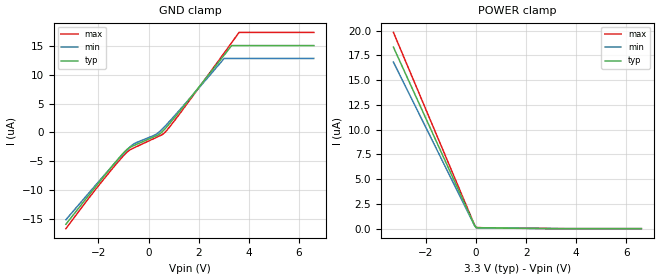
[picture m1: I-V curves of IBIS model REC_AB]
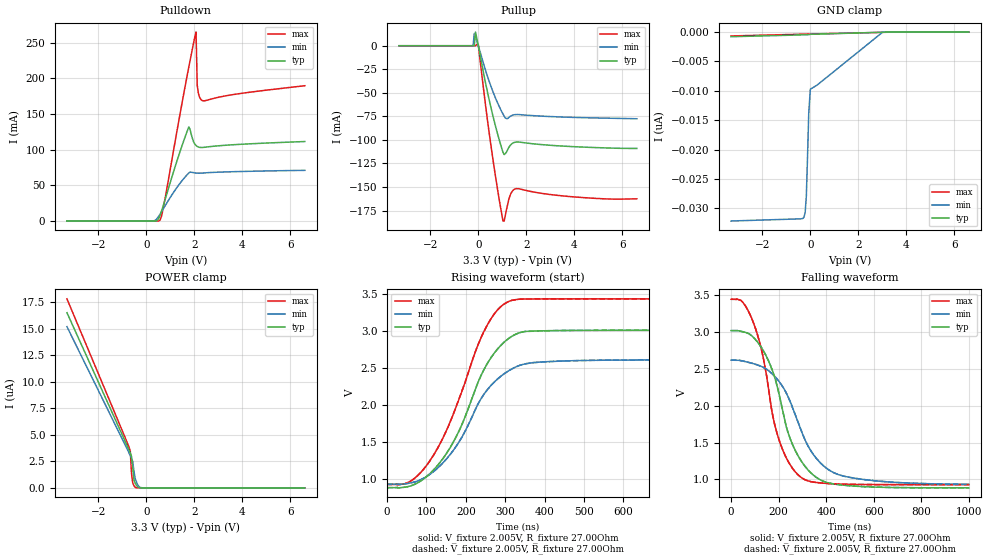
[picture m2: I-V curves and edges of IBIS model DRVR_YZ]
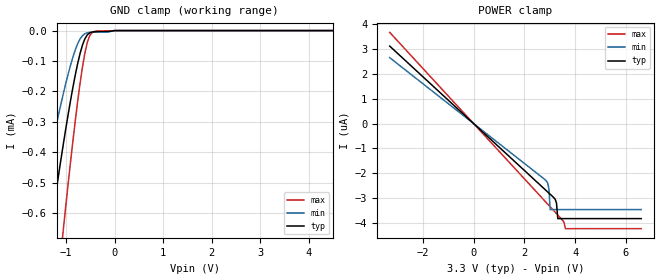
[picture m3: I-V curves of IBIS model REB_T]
| Texas Instruments Incorporated
| ISO35T ISOLATED 3.3V RS-485 TRANSCEIVER with Integrated Transformer Driver
| Marketing part#   Voltage Range   Package-type   #pins/pkg drawing
| ISO35TDW   3.0V - 3.6V   DW   16-pin
| ISO35TDWR   3.0V - 3.6V   DW   16-pin
[IBIS Ver]   4.0
[File name]   iso35t.ibs
[File Rev]   1.2
[Date]   02/28/2011
[Source]   TISPICE Simulations
   Texas Instruments Incorporated.
   Analog-eLab, HPA
   12500 TI Blvd
   Dallas, TX -75243
   For Support e-mail: elab_ibis@list.ti.com
[Notes]   Revision History
   Rev 1.0: 07/08/2008
   - Original model from Data Transmission Products Group
   Rev 1.1: 02/08/2011
   - file name changed from iso35.ibs to iso35_t.ibs
   - Updated header information
   - Updated all models with latest IBIS models generated from TISPICED
   - Pulldown/up non-monotonic warnings reflect true buffer behavior
   in TISPICED
   - Updated ccomp for all models as well
   - D1 and D2 are analog transformer driver pins that are outside
   the scope of IBIS 4.0 and hence are left as NCs
   - All the digtial buffer models are shared between ISO35 and ISO35T
   Rev 1.2: 02/28/2011
   - Removed ISO35 model from the file and renamed the file as ISO35T only
   - DRVR_YZ non-monotonicity is based on original
   simulations in TISPICED
[Disclaimer] This model is designed as an aid for customers of
 Texas Instruments. TI and its licensors and suppliers make no warranties,
 either expressed or implied, with respect to this  model, including the
 warranties of merchantability or fitness for a particular purpose.
 The model is provided solely on an "as is" basis. The entire risk as to
 its quality and performance is with the customer.
[Copyright] (C)Copyright 2011 Texas Instruments Incorporated.
   All rights reserved.
|   ISO35TDW  & ISO35TDWR
[Component]   ISO35TDW
[Manufacturer]  Texas Instruments Incorporated
[Package]   |16-pin DW package
|   typ   min   max
R_pkg   0.04229   0.019   0.0747
L_pkg   1.96583nH   1.3071nH   2.78nH
C_pkg   0.55243pF   0.366pF   0.8774pF
[Pin]   signal_name   model_name   R_pin   L_pin   C_pin
   1   D1   NC   0.01988  2.47032nH   0.87737pF
   2   D2   NC   0.01896  1.75378nH   0.75515pF
   3   GND1   GND   0.01119  1.36813nH   0.62214pF
   4   VCC1   POWER   0.01441  1.13364nH   0.53256pF
   5   R   OUT_R_T 0.02905  1.67358nH   0.55809pF
   6   REN   REB_T   0.03208  1.30711nH   0.39487pF
   7   DE   D_DE_T  0.03561  1.87226nH   0.60690pF
   8   D   D_DE_T  0.03804  2.78001nH   0.80551pF
   9   VCC2   POWER   0.02887  3.18832nH   2.5960pF
   10   GND2   GND   0.06791  2.86161nH   0.65609pF
   11   A   REC_AB  0.07468  2.23033nH   0.39167pF
   12   B   REC_AB  0.06522  2.01365nH   0.38729pF
   13   Z   DRVR_YZ 0.05893  1.87256nH   0.38126pF
   14   Y   DRVR_YZ 0.05043  1.68460nH   0.36601pF
   15   GND2   GND   0.03460  0.66170nH   3.0671pF
   16   GND2   GND   0.02304  3.19116nH   0.88927pF
[Diff_pin]   inv_pin   vdiff   tdelay_typ   tdelay_min   tdelay_max
| The 'A' pin is Diff_pin and the 'B' pin is the inv_pin
11   12   NA   0 0 0
14   13   0.200   0 0 0
[Pin Mapping] pulldown_ref pullup_ref gnd_clamp_ref power_clamp_ref |ext_ref
1   NC   NC
2   NC   NC
3   GND1BUS  NC
4   NC   VCC1BUS
5   GND1BUS  VCC1BUS  GND1BUS  VCC1BUS
6   NC   NC   GND1BUS  VCC1BUS
7   NC   NC   GND1BUS  VCC1BUS
8   NC   NC   GND1BUS  VCC1BUS
9   NC   VCC2BUS
10   GND2BUS  NC
11   NC   NC   GND2BUS  VCC2BUS
12   NC   NC   GND2BUS  VCC2BUS
13   GND2BUS  VCC2BUS  GND2BUS  VCC2BUS
14   GND2BUS  VCC2BUS  GND2BUS  VCC2BUS
15   GND2BUS  NC
16   GND2BUS  NC
| Models and submodels in the file (5): REC_AB (Input), DRVR_YZ (I/O), REB_T (Input), D_DE_T (Input), OUT_R_T (Output)
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|   Receiver Input / Model
[Model]   REC_AB
Model_type   Input
|Signals   A,B
Vinl   = 0.99V
Vinh   = 2.31V
|Rref_diff = 96k  |Input Diff resistance
|Cref_diff = 16pF |Input Diff capacitance
|Vdiff can be +/- 200mV and Common mode can be betweem -7V to 12V
|   typ   min   max
|   (typ PVT)   (Fast PVT)   (Slow PVT)
C_comp   0.2533pF   0.2533pF   0.2533pF
[Model Spec]
Vinl   0.99V   0.9V   1.08V
Vinh   2.31V   2.1V   2.52V
|   typ   min   max
[Temperature Range]   27.0   85   -40
[Voltage range]   3.3V   3.0V   3.6V
[GND Clamp]
|   Voltage   I(typ)   I(min)   I(max)
-3.3V     -15.94uA   -15.15uA   -16.71uA
-2.007V   -8.832uA   -8.611uA   -9.299uA
-912.1mV  -3.159uA   -3.267uA   -3.635uA
-563.8mV  -2.228uA   -1.938uA   -2.639uA
331.7mV   -534.5nA   -236.4nA   -822.3nA
480.9mV   -132.9nA   303.7nA    -516.7nA
679.9mV   743.7nA    1.182uA    128nA
1.327V    4.137uA    4.315uA    3.74uA
3.018V    13.42uA    12.84uA    13.79uA
3.317V    15.08uA    12.84uA    15.58uA
3.615V    15.08uA    12.84uA    17.37uA
6.6V      15.08uA    12.84uA    17.37uA
[POWER Clamp]
|  Voltage   I(typ)   I(min)   I(max)
-3.3V     18.32uA    16.82uA    19.81uA
-66.33mV  368.3nA    338nA      398.3nA
0V        101.5nA    93.2nA     NA
3.615V    0A         0A         0A
6.6V      0A         0A         0A
|   Driver YZ model
[Model]   DRVR_YZ
Model_type   I/O
| Signals   Y,Z
Vinl   = 0.99V
Vinh   = 2.31V
Vmeas   = 2.6V   |Reference voltage for timing measurements
Rref   = 27   |Note: 54 Ohm load; single-ended configuration
Vref   = 2.005V
|   Timing specification test load voltage
|Cref_diff = 50pF
|Rref_diff = 54Ohms
| variable   typ   min   max
| Y/Z  3-state   (typ PVT)   (Slow PVT)   (Fast PVT)
C_comp   30.536pF   30.533pF   31.925pF
| Y/Z high state   (typ PVT)   (Slow PVT)   (Fast PVT)
|C_comp   42.644pF   41.559pF   50.167pF
| Y/Z low state   (typ PVT)   (Fast PVT)   (Slow PVT)
|C_comp   48.779pF   38.475pF   54.688pF
[Model Spec]
Vref   2.005V   1.73V   2.528V
Vmeas   2.6V   2.2V   3.0V
Vinl   0.99V   0.9V   1.08V
Vinh   2.31V   2.1V   2.52V
|   typ   min   max
[Temperature Range]   27.0   85   -40
[Voltage range]   3.3V   3.0V   3.6V
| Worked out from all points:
|   slope of the pulldown table from 0 to 0.495 V, typ, clamps not added: 206 ohm
|   slope of the pullup table from 0 to 0.495 V, typ, clamps not added: 7.93 ohm
|   falling waveform, V_fixture 2.005V, R_fixture 27.00Ohm: 20-80 % time 124ns typ, 150ns min, 100ns max; typ from 3.01 V to 0.886 V
|   rising waveform, V_fixture 2.005V, R_fixture 27.00Ohm: 20-80 % time 111ns typ, 116ns min, 111ns max; typ from 0.886 V to 3.01 V
|   rising waveform, V_fixture 2.005V, R_fixture 27.00Ohm: 20-80 % time 111ns typ, 116ns min, 111ns max; typ from 0.886 V to 3.01 V
|   falling waveform, V_fixture 2.005V, R_fixture 27.00Ohm: 20-80 % time 124ns typ, 150ns min, 100ns max; typ from 3.01 V to 0.886 V
[Pulldown]
|   Voltage   I(typ)   I(min)   I(max)
-3.3V     -1.766pA   -150.1pA   -1.411pA
281.9mV   2.075uA    96.37uA    2.704nA
480.9mV   1.606mA    4.79mA     24.87uA
580.4mV   8.506mA    9.847mA    1.675mA
729.6mV   23.91mA    18.15mA    21.69mA
1.774V    132.1mA    67.49mA    216.4mA
1.973V    110.9mA    67.81mA    250.3mA
2.073V    105.9mA    67.31mA    265.2mA
2.123V    104.6mA    67.17mA    190.6mA
2.222V    103.4mA    67.09mA    173.5mA
2.322V    103.2mA    67.23mA    169.2mA
6.6V      111.5mA    71.11mA    189.8mA
[GND Clamp]
|   Voltage   I(typ)   I(min)   I(max)
-3.3V     -793.9pA   -32.13nA   -666.8pA
-414.6mV  -496.1pA   -31.76nA   -373.8pA
-315.1mV  -485.9pA   -31.7nA    -363.7pA
-265.3mV  -480.7pA   -31.51nA   -358.6pA
-215.6mV  -475.5pA   -30.72nA   -353.6pA
-165.8mV  -470pA     -27.89nA   -348.6pA
-116.1mV  -462.5pA   -21.21nA   -343.5pA
-66.33mV  -444.4pA   -13.88nA   -338.5pA
0V        -383.4pA   -9.718nA   -331.9pA
281.9mV   -355.3pA   -9.023nA   -306pA
3.018V    -34.94pA   0A         -54.81pA
6.6V      0A         0A         0A
[Pullup]
|   Voltage   I(typ)   I(min)   I(max)
-3.3V     2.176uA    1.898uA    2.571uA
-215.6mV  2.046uA    1.87uA     2.349uA
-165.8mV  2.035uA    13.06mA    2.343uA
-116.1mV  14.55mA    9.497mA    2.332uA
0V        333uA      106.1uA    1.39mA
480.9mV   -60.5mA    -39.81mA   -97.49mA
1.028V    -113.1mA   -72.45mA   -186.1mA
1.078V    -115.5mA   -74.75mA   -186mA
1.327V    -105.9mA   -75.02mA   -158.7mA
1.575V    -102.2mA   -73.06mA   -151.7mA
3.864V    -107mA     -75.99mA   -160.2mA
6.6V      -109mA     -77.51mA   -162.5mA
[POWER Clamp]
|   Voltage   I(typ)   I(min)   I(max)
-3.3V     16.5uA     15.18uA    17.8uA
-713.1mV  3.545uA    3.269uA    3.809uA
-663.3mV  3.278uA    3.03uA     3.448uA
-613.6mV  2.969uA    2.777uA    1.364uA
-563.8mV  1.935uA    2.476uA    483nA
-514.1mV  759.6nA    1.616uA    220.4nA
-464.3mV  464.5nA    906.1nA    56.28nA
-364.8mV  104.6nA    335.5nA    1.922nA
-315.1mV  31.05nA    149.1nA    812.5pA
-165.8mV  723.7pA    8.699nA    291.5pA
6.6V      0A         0A         0A
[Ramp]
R_load = 27.00Ohm
|   typ   min   max
dV/dt_r   1.277V/111.169ns   1.008V/115.508ns   1.505V/111.053ns
dV/dt_f   1.277V/123.529ns   1.008V/150.163ns   1.505V/100.109ns
[Falling Waveform]
V_fixture = 2.005V
V_fixture_min = 1.730V
V_fixture_max = 2.528V
R_fixture = 27.00Ohm
|   Time   V(typ)   V(min)   V(max)
0s        3.014V     2.614V     3.438V
73.3ns    2.975V     2.585V     3.275V
141.9ns   2.707V     2.506V     2.541V
173.6ns   2.476V     2.428V     1.891V
199.8ns   2.185V     2.335V     1.555V
239.5ns   1.636V     2.121V     1.248V
291.6ns   1.268V     1.688V     1.035V
360.8ns   1.023V     1.277V     957.5mV
452.4ns   930.1mV    1.065V     937.9mV
1us       886.5mV    933.5mV    930.1mV
[Rising Waveform]
V_fixture = 2.005V
V_fixture_min = 1.730V
V_fixture_max = 2.528V
R_fixture = 27.00Ohm
|   Time   V(typ)   V(min)   V(max)
0s        886.5mV    933.5mV    930.1mV
58.1ns    907.4mV    948.8mV    970.2mV
111.2ns   1.089V     1.077V     1.27V
175.1ns   1.571V     1.443V     1.977V
246.1ns   2.484V     2.15V      2.999V
276.7ns   2.736V     2.337V     3.266V
307.5ns   2.898V     2.462V     3.4V
346.9ns   2.994V     2.555V     3.436V
428.8ns   3.01V      2.595V     3.438V
1us       3.014V     2.614V     3.438V
[Rising Waveform]
V_fixture = 2.005V
V_fixture_min = 1.730V
V_fixture_max = 2.528V
R_fixture = 27.00Ohm
|   Time   V(typ)   V(min)   V(max)
0s        886.5mV    933.5mV    930.1mV
58.1ns    907.4mV    948.8mV    970.2mV
111.2ns   1.089V     1.077V     1.27V
175.1ns   1.571V     1.443V     1.977V
246.1ns   2.484V     2.15V      2.999V
276.7ns   2.736V     2.337V     3.266V
307.5ns   2.898V     2.462V     3.4V
347ns     2.995V     2.555V     3.436V
428.8ns   3.01V      2.595V     3.438V
1us       3.014V     2.614V     3.438V
[Falling Waveform]
V_fixture = 2.005V
V_fixture_min = 1.730V
V_fixture_max = 2.528V
R_fixture = 27.00Ohm
|   Time   V(typ)   V(min)   V(max)
0s        3.014V     2.614V     3.438V
73.3ns    2.975V     2.585V     3.275V
141.9ns   2.707V     2.506V     2.541V
173.6ns   2.476V     2.428V     1.891V
199.8ns   2.185V     2.335V     1.555V
239.5ns   1.636V     2.121V     1.248V
291.6ns   1.268V     1.688V     1.035V
360.8ns   1.023V     1.277V     957.5mV
452.4ns   930.1mV    1.065V     937.9mV
1us       886.5mV    933.5mV    930.1mV
|   Receiver Enable Model  ISO6277
[Model]   REB_T
Model_type   Input
|Signals   REB
Vinl   = 0.99V
Vinh   = 2.31V
|   typ   min   max
|ccomp   (typ PVT)   (Slow PVT)   (Fast PVT)
C_comp   0.25330759pF   0.25330759pF   0.25330760pF
[Model Spec]
Vinl   0.99V   0.9V   1.08V
Vinh   2.31V   2.1V   2.52V
|   typ   min   max
[Temperature Range]   27.0   85   -40
[Voltage range]   3.3V   3.0V   3.6V
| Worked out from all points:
|   GND clamp passes 1 mA (typ) near -1.62 V on its own axis
[GND Clamp]
|   Voltage   I(typ)   I(min)   I(max)
-3.3V     -3.149mA   -2.191mA   -4.612mA
-1.658V   -1.043mA   -672.3uA   -1.642mA
-1.609V   -983.6uA   -630.5uA   -1.557mA
-1.36V    -695.5uA   -428.5uA   -1.136mA
-1.31V    -639.8uA   -389.7uA   -1.053mA
-1.061V   -374.4uA   -208.2uA   -655.6uA
-812.6mV  -145.2uA   -62.95uA   -294.8uA
-713.1mV  -74.12uA   -27uA      -171.1uA
-613.6mV  -26.31uA   -10.23uA   -72.15uA
-514.1mV  -7.32uA    -5.94uA    -16.33uA
-364.8mV  -3.481uA   -5.062uA   -1.548uA
6.6V      0A         0A         0A
[POWER Clamp]
|   Voltage   I(typ)   I(min)   I(max)
-3.3V     3.123uA    2.656uA    3.676uA
2.819V    -2.667uA   -2.271uA   -3.14uA
2.919V    -2.762uA   -2.401uA   -3.251uA
2.968V    -2.809uA   -2.639uA   -3.307uA
3.018V    -2.856uA   -3.472uA   -3.362uA
3.217V    -3.063uA   -3.472uA   -3.584uA
3.267V    -3.216uA   -3.472uA   -3.639uA
3.317V    -3.837uA   -3.472uA   -3.694uA
3.565V    -3.837uA   -3.472uA   -3.994uA
3.615V    -3.837uA   -3.472uA   -4.242uA
6.6V      -3.837uA   -3.472uA   -4.242uA
